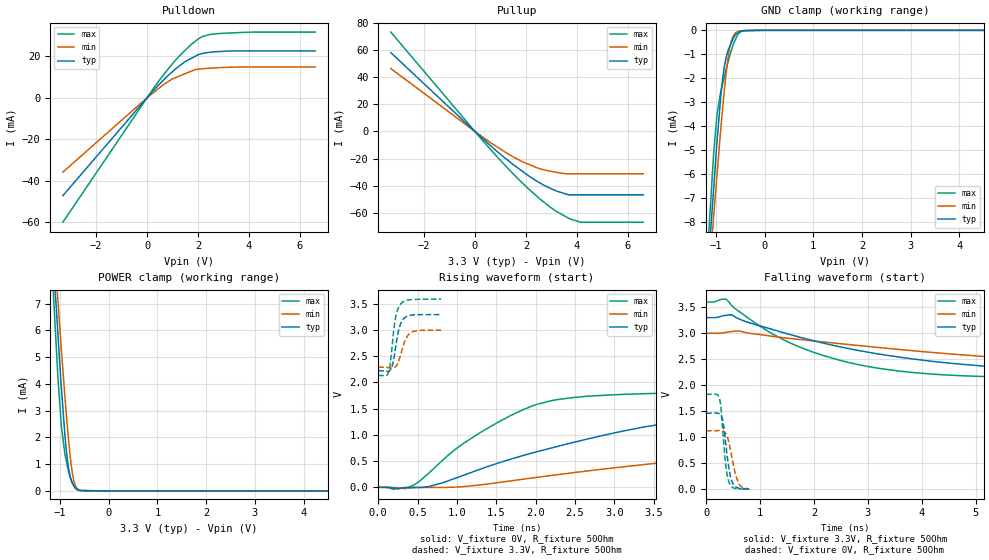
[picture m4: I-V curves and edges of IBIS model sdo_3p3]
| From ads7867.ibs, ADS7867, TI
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|   sdo_3p3 Model
[Model]   sdo_3p3
Model_type   3-state
Polarity   Non-Inverting
Vmeas = 1.65
Vref = 1.65
Cref = 2pF
Rref = 50
|   typ   min   max
|   (nom PVT)   (fast PVT)   (slow PVT)
|C_comp from frequency sweep method (F=1.7MHz)
|C_comp   1.803e-12   1.226e-12   3.012e-12
|ON state : BUFFER OUTPUT TURNED HIGH
|C_comp   1.803e-12   1.226e-12   3.012e-12
|OFF state: BUFFER IN HIGH IMPEDANCE
|C_comp   7.183e-13   7.101e-13   7.263e-13
|C_comp from LC tank measurement(L=1nH)
|Resonant Frequency(Hz)   6.650e+09   6.660e+09   6.550e+09
C_comp   5.734e-13   5.716e-13   5.910e-13
|ON state : BUFFER OUTPUT TURNED HIGH
|Resonant Frequency(Hz)   6.650e+09   6.660e+09   6.550e+09
|C_comp   5.734e-13   5.716e-13   5.910e-13
|OFF state: BUFFER IN HIGH IMPEDANCE
|Resonant Frequency(Hz)   6.760e+09   6.800e+09   6.730e+09
|C_comp   5.549e-13   5.483e-13   5.598e-13
| Where nom  PVT is Nominal Process, 3.3V, 27C
|   Fast PVT is Strong Process,  3.6V, -40C
|   Slow PVT is Weak Process,   3V, 87C
[Voltage Range]   3.3   3   3.6
|Ambient Temperature   25   85   -40
|Junction Temperature
[Temperature Range]   27   87   -40
[Pullup Reference]   3.3   3   3.6
[Pulldown Reference]   0   0   0
[Power Clamp Reference]   3.3   3   3.6
[GND Clamp Reference]   0   0   0
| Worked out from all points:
|   slope of the pulldown table from 0 to 0.495 V, typ, clamps not added: 73.9 ohm
|   slope of the pullup table from 0 to 0.495 V, typ, clamps not added: 58.1 ohm
|   GND clamp passes 1 mA (typ) near -0.77 V on its own axis
|   POWER clamp passes 1 mA (typ) near -0.84 V on its own axis
|   falling waveform, V_fixture 3.3V, R_fixture 50Ohm: 20-80 % time 3.21ns typ, 5.25ns min, 1.94ns max; typ from 3.3 V to 2.22 V
|   rising waveform, V_fixture 0V, R_fixture 50Ohm: 20-80 % time 2.26ns typ, 4.52ns min, 1.1ns max; typ from 0 V to 1.46 V
|   rising waveform, V_fixture 3.3V, R_fixture 50Ohm: 20-80 % time 79.5ps typ, 94.3ps min, 72.2ps max; typ from 2.22 V to 3.29 V
|   falling waveform, V_fixture 0V, R_fixture 50Ohm: 20-80 % time 110ps typ, 138ps min, 93.2ps max; typ from 1.46 V to 0.005 V
[Pulldown]
|   Voltage   I(typ)   I(min)   I(max)
-3.3V     -47.24mA   -35.9mA    -60.09mA
18mV      254.9uA    196.5uA    330.4uA
478.8mV   6.492mA    4.74mA     8.398mA
975mV     12.41mA    9.02mA     16.16mA
1.246V    15.19mA    10.4mA     19.94mA
1.706V    18.9mA     12.75mA    25.52mA
2.012V    20.87mA    13.85mA    28.47mA
2.167V    21.43mA    14.07mA    29.56mA
2.473V    21.99mA    14.32mA    30.62mA
2.934V    22.42mA    14.64mA    31.15mA
4.162V    22.64mA    14.87mA    31.75mA
6.6V      22.64mA    14.87mA    31.76mA
[GND Clamp]
|   Voltage   I(typ)   I(min)   I(max)
-3.3V     -80.51mA   -71.58mA   -94.81mA
-1.14V    -9.406mA   -10.26mA   -8.281mA
-1.099V   -8.14mA    -9.175mA   -6.921mA
-1.048V   -6.669mA   -7.822mA   -5.224mA
-975.6mV  -4.637mA   -6.024mA   -3.5mA
-897.6mV  -2.725mA   -4.082mA   -2.538mA
-828.3mV  -1.54mA    -2.548mA   -1.948mA
-756mV    -885.9uA   -1.242mA   -1.361mA
-687mV    -543.7uA   -477.4uA   -878.1uA
-537mV    -88.64uA   -36.72uA   -139.8uA
-133.2mV  -5.582uA   -36.76nA   0A
6.6V      0A         0A         0A
[Pullup]
|   Voltage   I(typ)   I(min)   I(max)
-3.3V     58.33mA    46.55mA    73.49mA
633mV     -10.85mA   -8.533mA   -13.77mA
1.26V     -20.86mA   -16.14mA   -26.65mA
1.86V     -29.4mA    -22.35mA   -38.07mA
2.475V    -37.26mA   -27.12mA   -48.71mA
2.934V    -41.81mA   -29.29mA   -55.64mA
3.175V    -43.82mA   -30.12mA   -58.86mA
3.683V    -46.85mA   -31.23mA   -64.25mA
4.133V    -46.85mA   -31.23mA   -67.01mA
6.6V      -46.85mA   -31.23mA   -67.06mA
[POWER Clamp]
|   Voltage   I(typ)   I(min)   I(max)
-3.3V     80.95mA    72.04mA    95.23mA
-1.134V   8.586mA    9.525mA    7.321mA
-1.096V   7.389mA    8.501mA    6.021mA
-1.048V   5.999mA    7.221mA    4.396mA
-972mV    3.859mA    5.273mA    2.414mA
-897.6mV  2.031mA    3.47mA     1.353mA
-861.3mV  1.347mA    2.662mA    1.037mA
-825mV    845uA      1.907mA    729uA
-747mV    288.3uA    673uA      284.7uA
-714mV    189.4uA    365uA      182.5uA
-648mV    64.61uA    86.45uA    39.38uA
6.6V      0A         0A         0A
[Ramp]
R_load = 50
|   typ   min   max
dV/dt_r   0.877427/2.25118e-09   0.673398/4.56945e-09   1.09564/1.10137e-09
dV/dt_f   0.647191/3.21256e-09   0.425148/5.24368e-09   0.880525/1.93443e-09
[Falling Waveform]
V_fixture = 3.3V
V_fixture_min = 3V
V_fixture_max = 3.6V
R_fixture = 50Ohm
|   Time   V(typ)   V(min)   V(max)
0s        3.3V       3V         3.6V
372ps     3.345V     3.017V     3.649V
632ps     3.265V     3.041V     3.404V
1.202ns   3.081V     2.945V     3.004V
2.152ns   2.815V     2.836V     2.579V
3.08ns    2.622V     2.738V     2.347V
4.193ns   2.461V     2.632V     2.215V
6.129ns   2.311V     2.489V     2.148V
9.656ns   2.236V     2.353V     2.133V
20ns      2.221V     2.291V     2.132V
[Rising Waveform]
V_fixture = 0V
V_fixture_min = 0V
V_fixture_max = 0V
R_fixture = 50Ohm
|   Time   V(typ)   V(min)   V(max)
0s        683.5pV    1.347nV    597.7pV
443ps     -3.788mV   -3.213mV   34.68mV
1.088ns   232.7mV    14.91mV    842.5mV
1.85ns    610.5mV    156.9mV    1.486V
2.194ns   747.4mV    225.3mV    1.65V
2.681ns   928.9mV    316.7mV    1.74V
3.854ns   1.261V     509.4mV    1.801V
5.257ns   1.392V     717.6mV    1.82V
8.766ns   1.453V     1.031V     1.826V
15.01ns   1.462V     1.114V     1.826V
[Rising Waveform]
V_fixture = 3.3V
V_fixture_min = 3V
V_fixture_max = 3.6V
R_fixture = 50Ohm
|   Time   V(typ)   V(min)   V(max)
0s        2.221V     2.29V      2.132V
131ps     2.213V     2.281V     2.2V
155ps     2.241V     2.275V     2.381V
178ps     2.314V     2.272V     2.706V
217ps     2.627V     2.295V     3.199V
253ps     2.951V     2.38V      3.408V
284ps     3.113V     2.519V     3.492V
351ps     3.249V     2.83V      3.561V
424ps     3.282V     2.957V     3.579V
799ps     3.292V     2.996V     3.589V
[Falling Waveform]
V_fixture = 0V
V_fixture_min = 0V
V_fixture_max = 0V
R_fixture = 50Ohm
|   Time   V(typ)   V(min)   V(max)
0s        1.462V     1.125V     1.826V
192ps     1.467V     1.128V     1.828V
247ps     1.453V     1.132V     1.754V
272ps     1.428V     1.131V     1.601V
304ps     1.347V     1.124V     1.199V
365ps     878.1mV    1.075V     466.2mV
433ps     344.5mV    855.5mV    119.9mV
498ps     110.8mV    512.2mV    34.21mV
591ps     26.55mV    148.3mV    11.3mV
799ps     5.422mV    10.95mV    4.957mV
